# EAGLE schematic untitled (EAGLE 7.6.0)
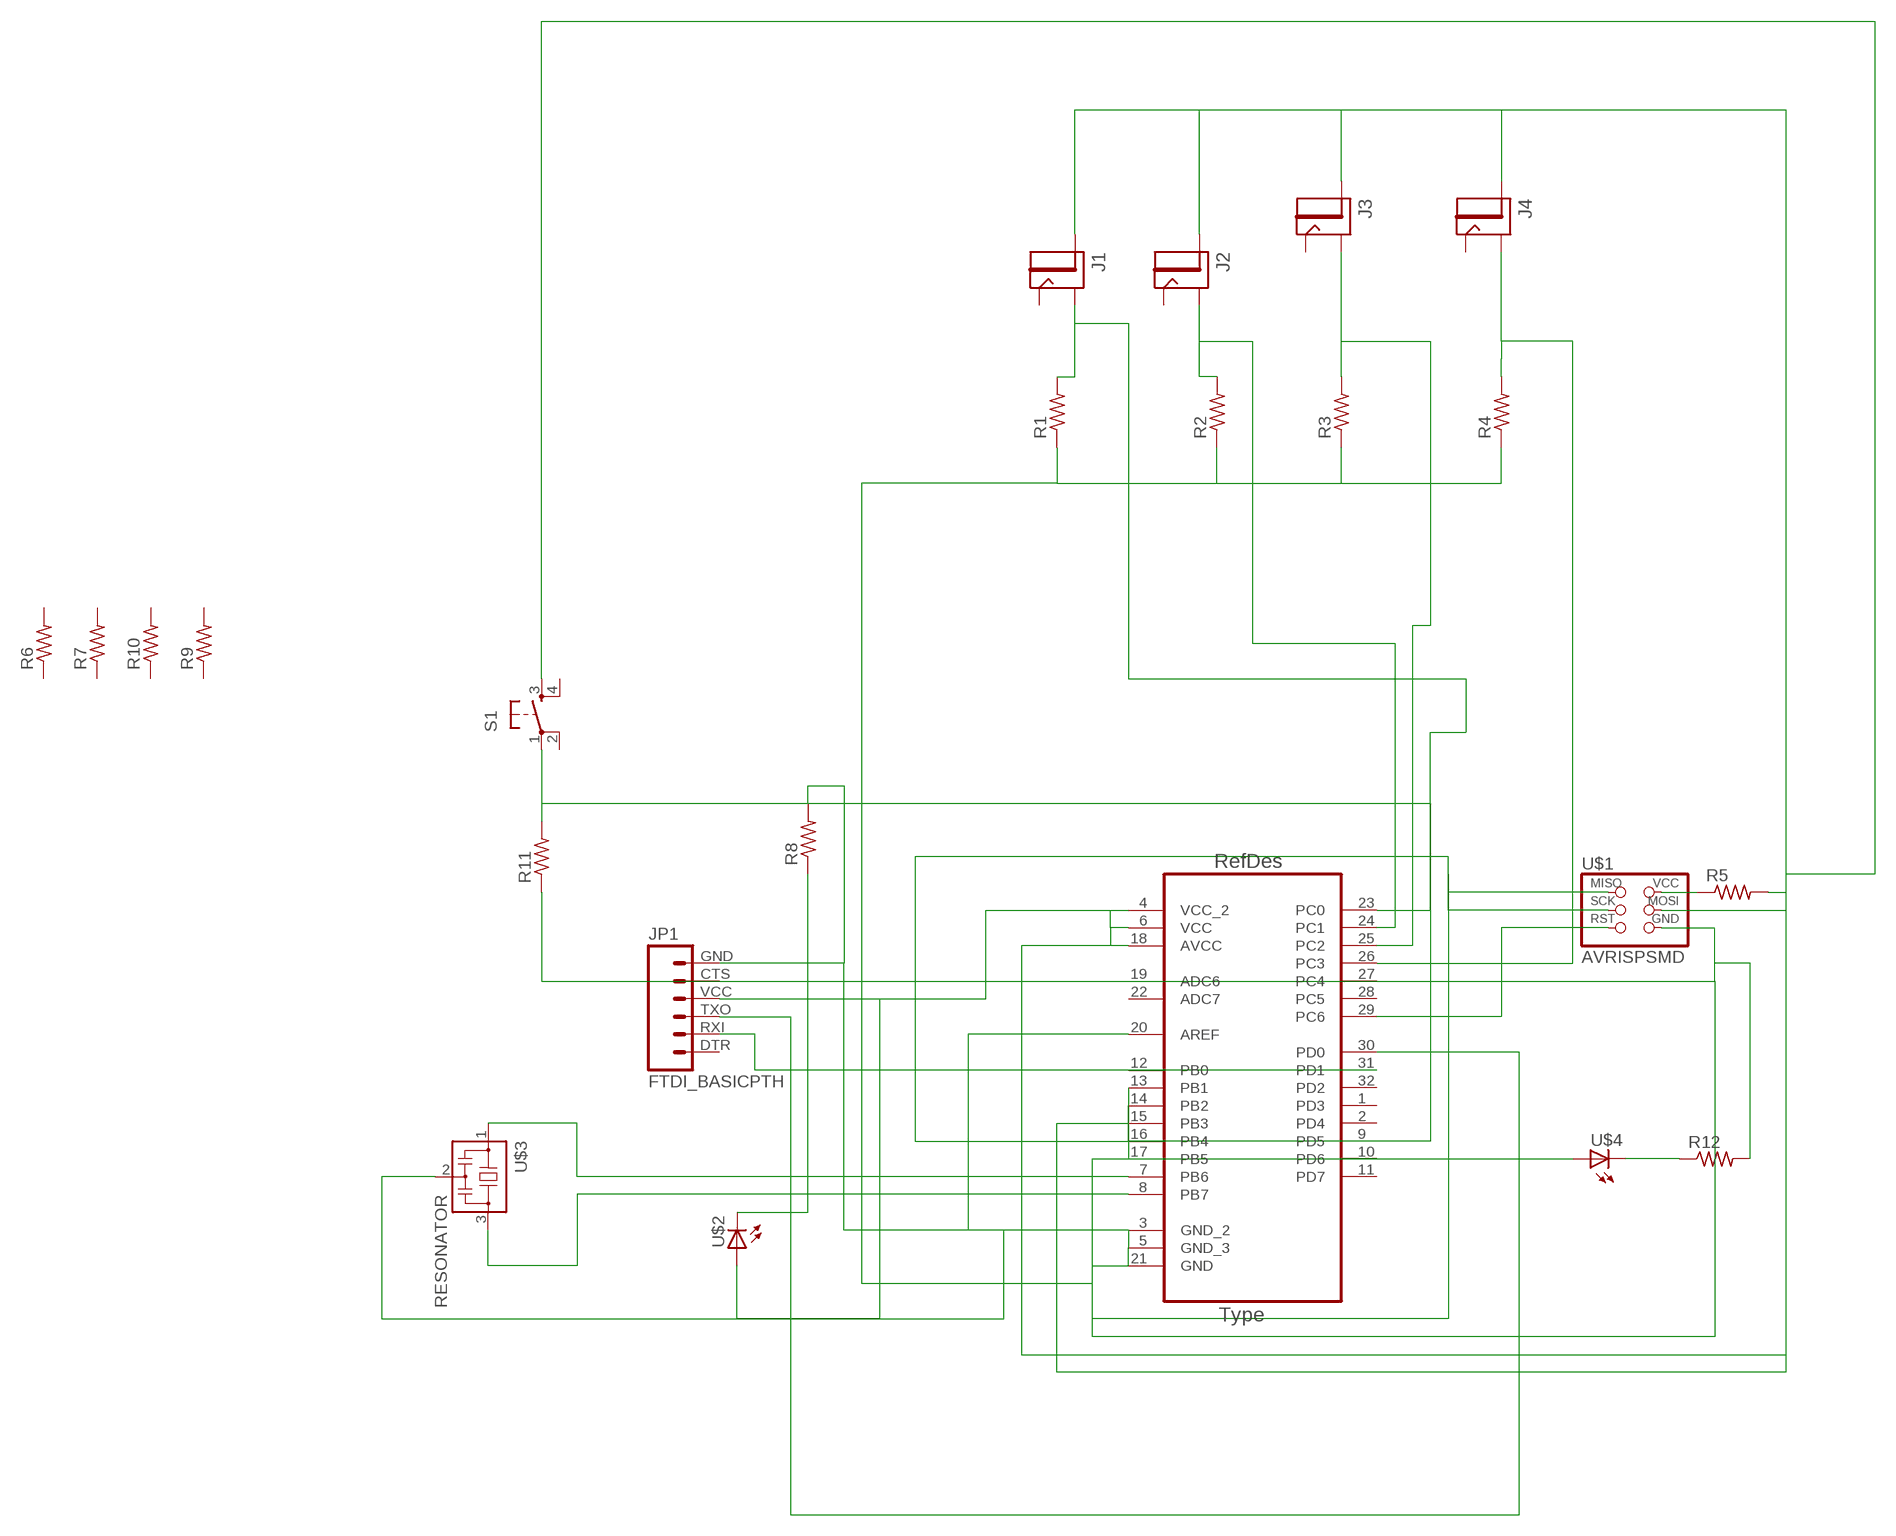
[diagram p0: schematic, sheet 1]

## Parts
J1  JACK.65MM  [JACK_.65MM]
J2  JACK.65MM  [JACK_.65MM]
J3  JACK.65MM  [JACK_.65MM]
J4  JACK.65MM  [JACK_.65MM]
JP1  FTDI_BASICPTH  [FTDI_BASIC]
R1  RES-US1206FAB  [R1206FAB]
R2  RES-US1206FAB  [R1206FAB]
R3  RES-US1206FAB  [R1206FAB]
R4  RES-US1206FAB  [R1206FAB]
R5  RES-US1206FAB  [R1206FAB]
R6  RES-US1206FAB  [R1206FAB]
R7  RES-US1206FAB  [R1206FAB]
R8  RES-US1206FAB  [R1206FAB]
R9  RES-US1206FAB  [R1206FAB]
R10  RES-US1206FAB  [R1206FAB]
R11  RES-US1206FAB  [R1206FAB]
R12  RES-US1206FAB  [R1206FAB]
S1  6MM_SWITCH6MM_SWITCH  [6MM_SWITCH]
U1  ATMEGA328P-AU  [QFP80P900X900X120-32N]
U$1  AVRISPSMD  [2X03SMD]
U$2  LED1206  [1206]
U$3  RESONATOR  [EFOBM]
U$4  LED1206  [1206]

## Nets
N$1: R5.1 U$1.2(VCC)
N$3: U1.15(PB3) U$1.4(MOSI)
N$4: U1.16(PB4) U$1.1(MISO)
N$5: U1.29(PC6) U$1.5(RST)
N$6: U1.17(PB5) U$1.3(SCK)
N$7: JP1.GND R1.1 R2.1 R3.1 R4.1 R8.2 R11.1 R12.2 U1.3(GND_2) U1.5(GND_3) U1.20(AREF) U1.21(GND) U$1.6(GND) U$3.2
N$8: J1.CONTACT(SHUNT) R1.2 U1.23(PC0)
N$9: J2.CONTACT(SHUNT) R2.2 U1.24(PC1)
N$10: J3.CONTACT(SHUNT) R3.2 U1.25(PC2)
N$11: J4.CONTACT(SHUNT) R4.2 U1.26(PC3)
N$13: J1.PIN J2.PIN J3.PIN J4.PIN JP1.VCC R5.2 S1.3(S) U1.4(VCC_2) U1.6(VCC) U1.18(AVCC) U$2.1(A)
N$14: JP1.TXO U1.30(PD0)
N$15: JP1.RXI U1.31(PD1)
N$16: R8.1 U$2.2(C)
N$17: U1.7(PB6) U$3.1
N$18: U1.8(PB7) U$3.3
N$19: R11.2 S1.1(P) U1.14(PB2)
N$20: R12.1 U$4.2(C)
N$21: U1.13(PB1) U$4.1(A)
Unconnected: J1.SHUNT(CONTACT) J2.SHUNT(CONTACT) J3.SHUNT(CONTACT) J4.SHUNT(CONTACT) JP1.CTS JP1.DTR R6.1 R6.2 R7.1 R7.2 R9.1 R9.2 R10.1 R10.2 S1.2(P1) S1.4(S1) U1.1(PD3) U1.2(PD4) U1.9(PD5) U1.10(PD6) U1.11(PD7) U1.12(PB0) U1.19(ADC6) U1.22(ADC7) U1.27(PC4) U1.28(PC5) U1.32(PD2)

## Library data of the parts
J1-J4 = fab:JACK
JP1 = SparkFun:FTDI_BASIC: FTDI Basic: 3.3V and 5V
R1-R12 = fab:RES-US: Resistor (US Symbol)
S1 = fab:6MM_SWITCH: OMRON SWITCH
U1 = Atmel-ATMEGA328P-AU:ATMEGA328P-AU; DESCRIPTION: 8-bit Microcontroller with In-System Programmable Flash; MPN: ATMEGA328P-AU; OC_FARNELL: 1715486; OC_NEWARK: 14R4631; PACKAGE: TQFP-32; SUPPLIER: Atmel
U$1 = fab:AVRISP
U$2 U$4 = FabLab:LED
U$3 = fab:RESONATOR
